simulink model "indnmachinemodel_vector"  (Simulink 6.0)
settings: Solver=ode4  StartTime=0  StopTime=1.2  FixedStep=1e-6  MaxStep=1e-4  RelTol=1e-3  AbsTol=1e-6
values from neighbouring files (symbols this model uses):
  fluxr = 0.2715    [PARAM.M]
  J = 0.0226    [PARAM.M]
  Lm = 4e-3    (= 0.004)    [PARAM.M]
  p = 4    [PARAM.M]
  Rr = .39    (= 0.39)    [PARAM.M]
  Rs = .19    (= 0.19)    [PARAM.M]
  Tr = Lr/Rr    (= 0.0117948717949)    [PARAM.M]
  Vd = 300    [PARAM.M]
  wb = 2*pi*fb    (= 628.318530718)    [PARAM.M]
  Xlr = wb*Llr    (= 0.376991118431)    [PARAM.M]
  Xls = wb*Lls    (= 0.131946891451)    [PARAM.M]
  Xmstar = 1/(1/Xls+1/Xm+1/Xlr)    (= 0.0940797800005)    [PARAM.M]
undefined symbols (not defined in the file or in its folder): magnitude
libraries: simulink x2

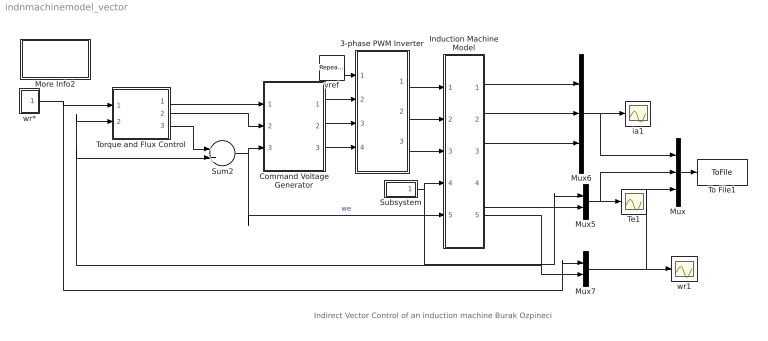
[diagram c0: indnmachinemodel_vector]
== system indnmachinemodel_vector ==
  note: Indirect Vector Control of an induction machine Burak Ozpineci
  3-phase PWM Inverter : Subsystem  PropExecContextAcrossSSBoundary=on
  Command Voltage Generator : Subsystem  PropExecContextAcrossSSBoundary=on
  Induction Machine Model : Subsystem  PropExecContextAcrossSSBoundary=on
  More Info2 : Subsystem  PropExecContextAcrossSSBoundary=on
  Mux : Mux  Inputs=3
  Mux5 : Mux  Inputs=2
  Mux6 : Mux  Inputs=3
  Mux7 : Mux  Inputs=2
  Subsystem : Subsystem  PropExecContextAcrossSSBoundary=on
  Sum2 : Sum
  Te1 : Scope
  To File1 : ToFile  Filename=iemdc2.mat  MatrixName=iemdc
  Torque and Flux Control : Subsystem  PropExecContextAcrossSSBoundary=on
  ia1 : Scope
  vref : simulink/Sources/Repeating Sequence  rep_seq_t=[0 25e-6 50e-6 75e-6 100e-6]  rep_seq_y=[0 1 0 -1 0]
  wr* : Subsystem  PropExecContextAcrossSSBoundary=on
  wr1 : Scope
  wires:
  Induction Machine Model/1(ia) -> Mux6/1
  Induction Machine Model/2(ib) -> Mux6/2
  Induction Machine Model/3(ic) -> Mux6/3
  vref/1 -> 3-phase PWM Inverter/1(vref)
  Torque and Flux Control/3(wsl) -> Sum2/1
  wr*/1(wr*) -> Torque and Flux Control/1(wr*), Mux7/1
  Sum2/1 -> Command Voltage Generator/3(we), Induction Machine Model/5(we)  "we"
  Torque and Flux Control/1(vqs*) -> Command Voltage Generator/1(vqs*)
  Torque and Flux Control/2(vds*) -> Command Voltage Generator/2(vds*)
  Command Voltage Generator/1(vao*) -> 3-phase PWM Inverter/2(vao*)
  Command Voltage Generator/2(vbo*) -> 3-phase PWM Inverter/3(vbo*)
  Command Voltage Generator/3(vco*) -> 3-phase PWM Inverter/4(vco*)
  3-phase PWM Inverter/3(vco) -> Induction Machine Model/3(vco)
  3-phase PWM Inverter/2(vbo) -> Induction Machine Model/2(vbo)
  3-phase PWM Inverter/1(vao) -> Induction Machine Model/1(vao)
  Mux6/1 -> Mux/1, ia1/1
  Induction Machine Model/4(Te) -> Mux5/2
  Mux5/1 -> Mux/2, Te1/1
  Induction Machine Model/5(wr) -> Torque and Flux Control/2(wr), Sum2/2, Mux7/2
  Mux7/1 -> wr1/1, Mux/3
  Subsystem/1(Tl) -> Induction Machine Model/4(Tl), Mux5/1
  Mux/1 -> To File1/1

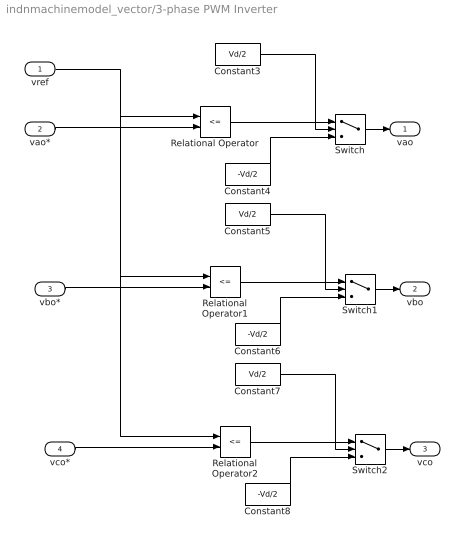
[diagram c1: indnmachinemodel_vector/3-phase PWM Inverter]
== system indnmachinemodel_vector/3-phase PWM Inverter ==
  vref : Inport  LatchInput=off
  vao* : Inport  Port=2  LatchInput=off
  vbo* : Inport  Port=3  LatchInput=off
  vco* : Inport  Port=4  LatchInput=off
  Constant3 : Constant  Value=Vd/2
  Constant4 : Constant  Value=-Vd/2
  Constant5 : Constant  Value=Vd/2
  Constant6 : Constant  Value=-Vd/2
  Constant7 : Constant  Value=Vd/2
  Constant8 : Constant  Value=-Vd/2
  Relational Operator : RelationalOperator  Operator=<=
  Relational Operator1 : RelationalOperator  Operator=<=
  Relational Operator2 : RelationalOperator  Operator=<=
  Switch : Switch  Threshold=0.5
  Switch1 : Switch  Threshold=0.5
  Switch2 : Switch  Threshold=0.5
  vao : Outport
  vbo : Outport  Port=2
  vco : Outport  Port=3
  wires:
  vao*/1 -> Relational Operator/2
  Switch/1 -> vao/1
  Constant4/1 -> Switch/3
  Constant3/1 -> Switch/1
  Relational Operator/1 -> Switch/2
  vbo*/1 -> Relational Operator1/2
  Switch1/1 -> vbo/1
  Constant6/1 -> Switch1/3
  Constant5/1 -> Switch1/1
  vco*/1 -> Relational Operator2/2
  Switch2/1 -> vco/1
  Constant8/1 -> Switch2/3
  Constant7/1 -> Switch2/1
  Relational Operator2/1 -> Switch2/2
  vref/1 -> Relational Operator/1, Relational Operator1/1, Relational Operator2/1
  Relational Operator1/1 -> Switch1/2

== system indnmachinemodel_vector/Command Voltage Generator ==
  vqs* : Inport  LatchInput=off
  vds* : Inport  Port=2  LatchInput=off
  we : Inport  Port=3  LatchInput=off
  Estimator1 : Subsystem  PropExecContextAcrossSSBoundary=on
  Syn-abc3 : Subsystem  PropExecContextAcrossSSBoundary=on
  unit vectors : Subsystem  PropExecContextAcrossSSBoundary=on
  vao* : Outport
  vbo* : Outport  Port=2
  vco* : Outport  Port=3
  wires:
  Syn-abc3/1(vao*) -> vao*/1
  unit vectors/1(cos(theta-e)) -> Syn-abc3/3(cos(theta-e))
  unit vectors/2(sin(theta-e)) -> Syn-abc3/4(sin(theta-e))
  Estimator1/1(theta-e) -> unit vectors/1(theta-e)
  we/1 -> Estimator1/1(we)
  vds*/1 -> Syn-abc3/2(vds)
  vqs*/1 -> Syn-abc3/1(vqs)
  Syn-abc3/2(vbo*) -> vbo*/1
  Syn-abc3/3(vco*) -> vco*/1

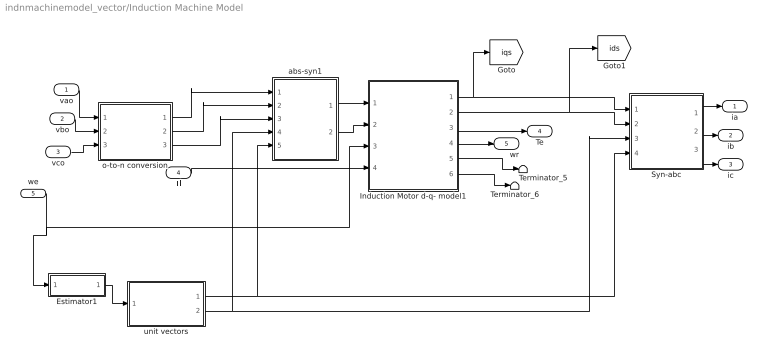
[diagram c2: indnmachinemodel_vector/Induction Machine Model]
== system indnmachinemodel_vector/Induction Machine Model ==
  vao : Inport  LatchInput=off
  vbo : Inport  Port=2  LatchInput=off
  vco : Inport  Port=3  LatchInput=off
  Tl : Inport  Port=4  LatchInput=off
  we : Inport  Port=5  LatchInput=off
  Estimator1 : Subsystem  PropExecContextAcrossSSBoundary=on
  Induction Motor d-q- model1 : Subsystem  PropExecContextAcrossSSBoundary=on
  Syn-abc : Subsystem  PropExecContextAcrossSSBoundary=on
  Terminator_5 : Terminator
  Terminator_6 : Terminator
  abs-syn1 : Subsystem  PropExecContextAcrossSSBoundary=on
  o-to-n conversion : Subsystem  PropExecContextAcrossSSBoundary=on
  unit vectors : Subsystem  PropExecContextAcrossSSBoundary=on
  ia : Outport
  ib : Outport  Port=2
  ic : Outport  Port=3
  Te : Outport  Port=4
  wr : Outport  Port=5
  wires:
  we/1 -> Induction Motor d-q- model1/3(we), Estimator1/1(we)
  Estimator1/1(theta-e) -> unit vectors/1(theta-e)
  Induction Motor d-q- model1/6("iqr ") -> Terminator_6/1
  Tl/1 -> Induction Motor d-q- model1/4(Tl)
  Syn-abc/2(ib) -> ib/1
  Syn-abc/3(ic) -> ic/1
  Induction Motor d-q- model1/5("idr ") -> Terminator_5/1
  Syn-abc/1(ia) -> ia/1
  Induction Motor d-q- model1/3("Te ") -> Te/1
  Induction Motor d-q- model1/4("wr ") -> wr/1
  vao/1 -> o-to-n conversion/1(vao)
  vbo/1 -> o-to-n conversion/2(vbo)
  vco/1 -> o-to-n conversion/3(vco)
  unit vectors/1(sin(theta-e)) -> Syn-abc/4(sin(theta-e)), abs-syn1/5(sin(theta-e))
  unit vectors/2(cos(theta-e)) -> Syn-abc/3(cos(theta-e)), abs-syn1/4(cos(theta-e))
  Induction Motor d-q- model1/2("ids ") -> Syn-abc/2(ids), [ids]
  Induction Motor d-q- model1/1("iqs ") -> [iqs], Syn-abc/1(iqs)
  o-to-n conversion/1(van) -> abs-syn1/1(van)
  o-to-n conversion/2(vbn) -> abs-syn1/2(vbn)
  o-to-n conversion/3(vcn) -> abs-syn1/3(vcn)
  abs-syn1/2(vds) -> Induction Motor d-q- model1/2(vds)
  abs-syn1/1(vqs) -> Induction Motor d-q- model1/1(vqs)

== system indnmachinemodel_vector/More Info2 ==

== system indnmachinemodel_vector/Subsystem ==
  Step2 : Step  Time=.8  After=20  SampleTime=0
  Step3 : Step  After=-10  SampleTime=0
  Step4 : Step  Time=30  After=0  SampleTime=0
  Sum1 : Sum  Inputs=|+++
  Tl : Outport
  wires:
  Step3/1 -> Sum1/2
  Step2/1 -> Sum1/1
  Step4/1 -> Sum1/3
  Sum1/1 -> Tl/1

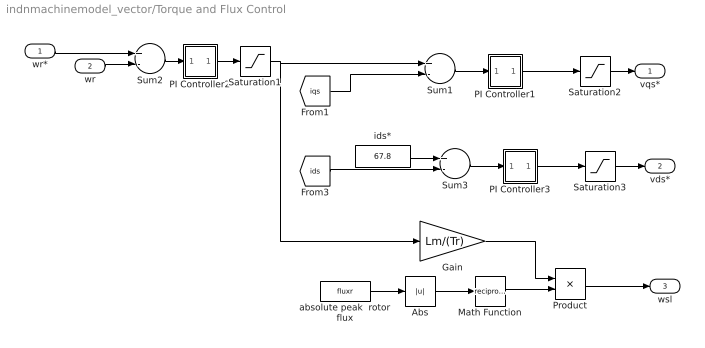
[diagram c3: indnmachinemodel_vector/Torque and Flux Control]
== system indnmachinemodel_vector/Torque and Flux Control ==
  wr* : Inport  LatchInput=off
  wr : Inport  Port=2  LatchInput=off
  Abs : Abs
  Gain : Gain  Gain=Lm/(Tr)
  Math Function : Math  Operator=reciprocal
  PI Controller1 : Subsystem  PropExecContextAcrossSSBoundary=on  mask(PI Controller){P=10000, I=100}
      mask prompts: P "Proportional:"; I "Integral:"
      mask help: Enter expressions for proportional, integral, and derivative terms. P+I/s
  PI Controller2 : Subsystem  PropExecContextAcrossSSBoundary=on  mask(PI Controller){P=500, I=1}
      mask prompts: P "Proportional:"; I "Integral:"
      mask help: Enter expressions for proportional, integral, and derivative terms. P+I/s
  PI Controller3 : Subsystem  PropExecContextAcrossSSBoundary=on  mask(PI Controller){P=1000, I=100}
      mask prompts: P "Proportional:"; I "Integral:"
      mask help: Enter expressions for proportional, integral, and derivative terms. P+I/s
  Product : Product
  Saturation1 : Saturate  UpperLimit=500  LowerLimit=-500
  Saturation2 : Saturate  UpperLimit=1  LowerLimit=-1
  Saturation3 : Saturate  UpperLimit=1  LowerLimit=-1
  Sum1 : Sum  Inputs=+-
  Sum2 : Sum  Inputs=+-
  Sum3 : Sum  Inputs=+-
  absolute peak  rotor flux : Constant  Value=fluxr
  ids* : Constant  Value=67.8
  vqs* : Outport  InitialOutput=0
  vds* : Outport  Port=2  InitialOutput=0
  wsl : Outport  Port=3  InitialOutput=0
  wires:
  absolute peak  rotor flux/1 -> Abs/1
  Gain/1 -> Product/1
  Abs/1 -> Math Function/1
  Math Function/1 -> Product/2
  wr/1 -> Sum2/2
  Sum2/1 -> PI Controller2/1(e)
  wr*/1 -> Sum2/1
  Product/1 -> wsl/1
  Sum1/1 -> PI Controller1/1(e)
  PI Controller2/1(m) -> Saturation1/1
  PI Controller1/1(m) -> Saturation2/1
  Saturation2/1 -> vqs*/1
  Saturation3/1 -> vds*/1
  Sum3/1 -> PI Controller3/1(e)
  PI Controller3/1(m) -> Saturation3/1
  [iqs] -> Sum1/2
  ids*/1 -> Sum3/1
  [ids] -> Sum3/2
  Saturation1/1 -> Gain/1, Sum1/1

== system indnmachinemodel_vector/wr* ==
  Repeating Sequence : simulink/Sources/Repeating Sequence  rep_seq_t=[0 .15 .35 .4 .55 .6 10]  rep_seq_y=[0 .8*wb .8*wb .50*wb .50*wb .65*wb .65*wb]
  wr* : Outport
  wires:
  Repeating Sequence/1 -> wr*/1

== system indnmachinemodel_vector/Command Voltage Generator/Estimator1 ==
  we : Inport  LatchInput=off
  Constant : Constant  Value=2*pi
  Integrator : Integrator  InitialCondition=pi/6
  Math Function3 : Math  Operator=mod
  theta-e : Outport
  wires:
  Math Function3/1 -> theta-e/1
  Integrator/1 -> Math Function3/1
  Constant/1 -> Math Function3/2
  we/1 -> Integrator/1

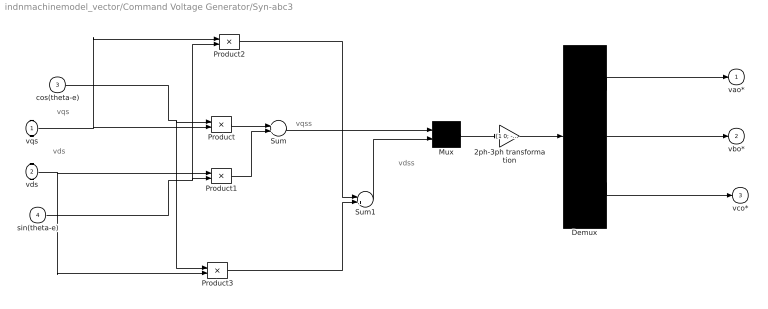
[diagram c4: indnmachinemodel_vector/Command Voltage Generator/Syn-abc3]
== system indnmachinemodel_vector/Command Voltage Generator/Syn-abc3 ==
  note: vqss
  note: vqs
  note: vdss
  note: vds
  vqs : Inport  LatchInput=off
  vds : Inport  Port=2  LatchInput=off
  cos(theta-e) : Inport  Port=3  LatchInput=off
  sin(theta-e) : Inport  Port=4  LatchInput=off
  2ph-3ph transformation : Gain  Gain="[1 0; -1/2 -sqrt(3)/2;  -1/2 sqrt(3)/2]"  Multiplication=Matrix(K*u)
  Demux : Demux  Outputs=3
  Mux : Mux  Inputs=2
  Product{,1..3} (4 alike) : Product
  Sum : Sum
  Sum1 : Sum  Inputs=-+
  vao* : Outport
  vbo* : Outport  Port=2
  vco* : Outport  Port=3
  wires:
  2ph-3ph transformation/1 -> Demux/1
  Sum1/1 -> Mux/2
  Product/1 -> Sum/1
  Product1/1 -> Sum/2
  sin(theta-e)/1 -> Product2/2, Product1/2
  cos(theta-e)/1 -> Product3/1, Product/1
  Product3/1 -> Sum1/2
  Product2/1 -> Sum1/1
  Mux/1 -> 2ph-3ph transformation/1
  vds/1 -> Product3/2, Product1/1
  vqs/1 -> Product2/1, Product/2
  Demux/1 -> vao*/1
  Demux/2 -> vbo*/1
  Demux/3 -> vco*/1
  Sum/1 -> Mux/1

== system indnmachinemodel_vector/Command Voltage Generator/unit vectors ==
  theta-e : Inport  LatchInput=off
  Trigonometric Function : Trigonometry
  Trigonometric Function1 : Trigonometry  Operator=cos
  cos(theta-e) : Outport
  sin(theta-e) : Outport  Port=2
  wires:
  Trigonometric Function/1 -> sin(theta-e)/1
  Trigonometric Function1/1 -> cos(theta-e)/1
  theta-e/1 -> Trigonometric Function1/1, Trigonometric Function/1

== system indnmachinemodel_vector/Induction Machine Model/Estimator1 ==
  we : Inport  LatchInput=off
  Constant : Constant  Value=2*pi
  Integrator : Integrator  InitialCondition=0.01
  Math Function3 : Math  Operator=mod
  theta-e : Outport
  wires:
  we/1 -> Integrator/1
  Constant/1 -> Math Function3/2
  Integrator/1 -> Math Function3/1
  Math Function3/1 -> theta-e/1

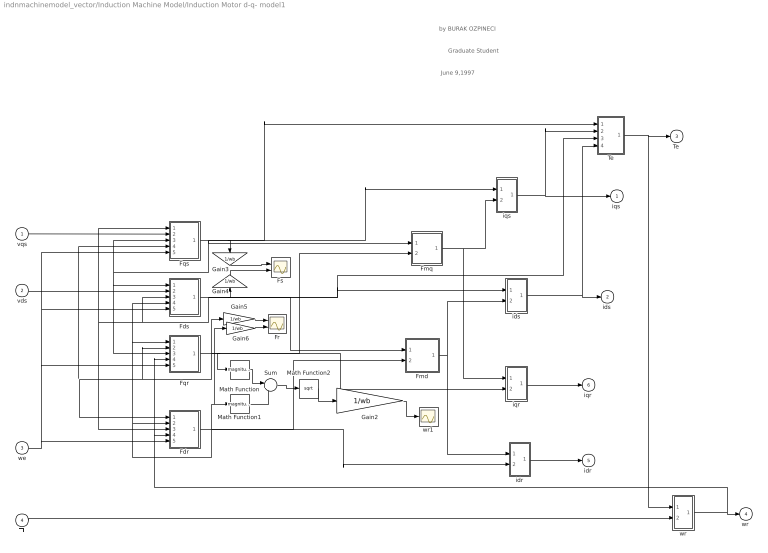
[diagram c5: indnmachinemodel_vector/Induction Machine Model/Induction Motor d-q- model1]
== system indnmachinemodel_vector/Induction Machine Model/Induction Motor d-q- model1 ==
  note: by BURAK OZPINECI
  note: Graduate Student
  note: June 9,1997
  vqs : Inport  LatchInput=off
  vds : Inport  Port=2  LatchInput=off
  we : Inport  Port=3  LatchInput=off
  Tl : Inport  Port=4  LatchInput=off
  Fdr : Subsystem  PropExecContextAcrossSSBoundary=on
  Fds : Subsystem  PropExecContextAcrossSSBoundary=on
  Fmd : Subsystem  PropExecContextAcrossSSBoundary=on
  Fmq : Subsystem  PropExecContextAcrossSSBoundary=on
  Fqr : Subsystem  PropExecContextAcrossSSBoundary=on
  Fqs : Subsystem  PropExecContextAcrossSSBoundary=on
  Fr : Scope  NumInputPorts=2
  Fs : Scope  NumInputPorts=2
  Gain2 : Gain  Gain=1/wb
  Gain3 : Gain  Orientation=down  Gain=1/wb
  Gain4 : Gain  Orientation=up  Gain=1/wb
  Gain5 : Gain  Gain=1/wb
  Gain6 : Gain  Gain=1/wb
  Math Function : Math  Operator=magnitude^2
  Math Function1 : Math  Operator=magnitude^2
  Math Function2 : Math  Operator=sqrt
  Sum : Sum  Inputs=|++
  Te : Subsystem  PropExecContextAcrossSSBoundary=on
  idr : Subsystem  PropExecContextAcrossSSBoundary=on
  ids : Subsystem  PropExecContextAcrossSSBoundary=on
  iqr : Subsystem  PropExecContextAcrossSSBoundary=on
  iqs : Subsystem  PropExecContextAcrossSSBoundary=on
  wr : Subsystem  PropExecContextAcrossSSBoundary=on
  wr1 : Scope
  "iqs " : Outport
  "ids " : Outport  Port=2
  "Te " : Outport  Port=3
  "wr " : Outport  Port=4
  "idr " : Outport  Port=5
  "iqr " : Outport  Port=6
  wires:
  Fdr/1("Fdr ") -> idr/2(Fdr), Fdr/2(Fdr), Fqr/1(Fdr), Fds/4(Fdr), Fmd/2(Fdr), Math Function1/1, Gain6/1
  we/1 -> Fqs/5(we), Fds/5(we), Fqr/5(we), Fdr/5(we)
  wr/1(wr) -> "wr "/1, Fqr/4(wr), Fdr/4(wr)
  vqs/1 -> Fqs/2(Vqs)
  vds/1 -> Fds/2(Vds)
  Tl/1 -> wr/2(Tl)
  Fqs/1("Fqs ") -> Fqs/3(Fqs), Fqr/3(Fqs), Fds/1(Fqs), Fmq/1(Fqs), iqs/1(Fqs), Te/1(Fqs), Gain3/1
  Fqr/1("Fqr ") -> Fqr/2(Fqr), Fqs/4(Fqr), Fdr/1(Fqr), Fmq/2(Fqr), Math Function/1, iqr/2(Fqr), Gain5/1
  Fds/1("Fds ") -> Fds/3(Fds), Fqs/1(Fds), Fdr/3(Fds), Fmd/1(Fds), ids/1(Fds), Te/3(Fds), Gain4/1
  iqr/1(iqr) -> "iqr "/1
  Fmq/1(Fmq) -> iqs/2(Fmq), iqr/1(Fmq)
  idr/1(idr) -> "idr "/1
  Fmd/1(Fmd) -> ids/2(Fmd), idr/1(Fmd)
  Te/1(Te) -> "Te "/1, wr/1(Te)
  ids/1(ids) -> "ids "/1, Te/4(ids)
  iqs/1(iqs) -> "iqs "/1, Te/2(iqs)
  Math Function/1 -> Sum/1
  Math Function1/1 -> Sum/2
  Sum/1 -> Math Function2/1
  Math Function2/1 -> Gain2/1
  Gain2/1 -> wr1/1
  Gain3/1 -> Fs/1
  Gain4/1 -> Fs/2
  Gain5/1 -> Fr/1
  Gain6/1 -> Fr/2

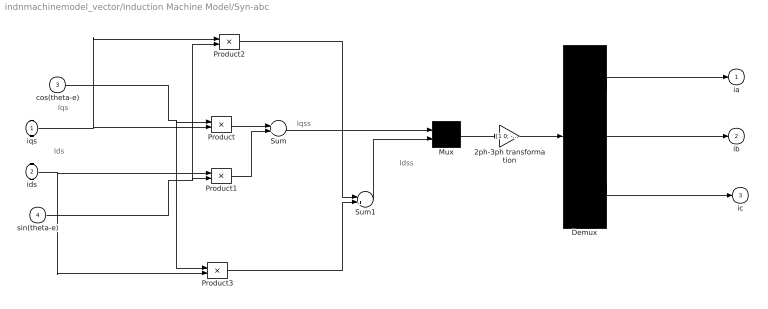
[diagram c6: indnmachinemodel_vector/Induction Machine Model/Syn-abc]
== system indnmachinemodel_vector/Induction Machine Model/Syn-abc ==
  note: Iqss
  note: Iqs
  note: Idss
  note: Ids
  iqs : Inport  LatchInput=off
  ids : Inport  Port=2  LatchInput=off
  cos(theta-e) : Inport  Port=3  LatchInput=off
  sin(theta-e) : Inport  Port=4  LatchInput=off
  2ph-3ph transformation : Gain  Gain="[1 0; -1/2 -sqrt(3)/2;  -1/2 sqrt(3)/2]"  Multiplication=Matrix(K*u)
  Demux : Demux  Outputs=3
  Mux : Mux  Inputs=2
  Product{,1..3} (4 alike) : Product
  Sum : Sum
  Sum1 : Sum  Inputs=-+
  ia : Outport
  ib : Outport  Port=2
  ic : Outport  Port=3
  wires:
  2ph-3ph transformation/1 -> Demux/1
  Sum1/1 -> Mux/2
  Sum/1 -> Mux/1
  Product/1 -> Sum/1
  Product1/1 -> Sum/2
  sin(theta-e)/1 -> Product2/2, Product1/2
  cos(theta-e)/1 -> Product3/1, Product/1
  Product3/1 -> Sum1/2
  Product2/1 -> Sum1/1
  Mux/1 -> 2ph-3ph transformation/1
  ids/1 -> Product3/2, Product1/1
  iqs/1 -> Product2/1, Product/2
  Demux/1 -> ia/1
  Demux/2 -> ib/1
  Demux/3 -> ic/1

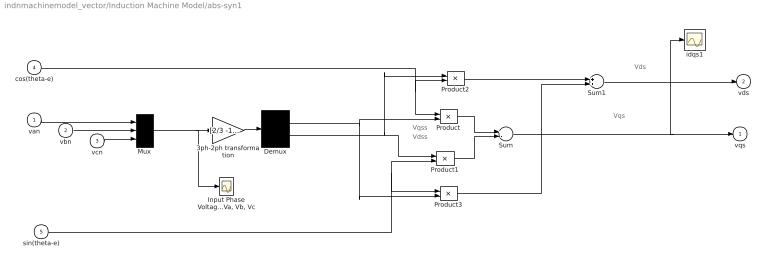
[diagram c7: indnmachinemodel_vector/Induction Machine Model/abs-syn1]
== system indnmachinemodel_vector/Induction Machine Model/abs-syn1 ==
  note: Vqs
  note: Vds
  note: Vqss
  note: Vdss
  van : Inport  LatchInput=off
  vbn : Inport  Port=2  LatchInput=off
  vcn : Inport  Port=3  LatchInput=off
  cos(theta-e) : Inport  Port=4  LatchInput=off
  sin(theta-e) : Inport  Port=5  LatchInput=off
  3ph-2ph transformation : Gain  Gain=[2/3 -1/3 -1/3;0 -1/sqrt(3) 1/sqrt(3)]  Multiplication=Matrix(K*u)
  Demux : Demux  Outputs=2
  "Input Phase Voltages Va, Vb, Vc" : Scope
  Mux : Mux  Inputs=3
  Product{,1..3} (4 alike) : Product
  Sum : Sum  Inputs=+-
  Sum1 : Sum
  idqs1 : Scope
  vqs : Outport
  vds : Outport  Port=2
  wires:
  cos(theta-e)/1 -> Product2/2, Product/1
  sin(theta-e)/1 -> Product3/1, Product1/2
  Demux/1 -> Product3/2, Product/2
  van/1 -> Mux/1
  Demux/2 -> Product1/1, Product2/1
  vbn/1 -> Mux/2
  Product3/1 -> Sum1/2
  Product2/1 -> Sum1/1
  Sum/1 -> idqs1/1, vqs/1
  Sum1/1 -> vds/1
  Product1/1 -> Sum/2
  Mux/1 -> 3ph-2ph transformation/1, "Input Phase Voltages Va, Vb, Vc"/1
  vcn/1 -> Mux/3
  Product/1 -> Sum/1
  3ph-2ph transformation/1 -> Demux/1

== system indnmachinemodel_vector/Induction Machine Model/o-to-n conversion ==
  vao : Inport  LatchInput=off
  vbo : Inport  Port=2  LatchInput=off
  vco : Inport  Port=3  LatchInput=off
  Demux : Demux  Outputs=3
  Matrix Gain : Gain  Gain=[2/3 -1/3 -1/3; -1/3 2/3 -1/3; -1/3 -1/3 2/3]  Multiplication=Matrix(K*u)
  Mux : Mux  Inputs=3
  van : Outport
  vbn : Outport  Port=2
  vcn : Outport  Port=3
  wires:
  Demux/3 -> vcn/1
  Demux/2 -> vbn/1
  Demux/1 -> van/1
  vco/1 -> Mux/3
  vbo/1 -> Mux/2
  vao/1 -> Mux/1
  Matrix Gain/1 -> Demux/1
  Mux/1 -> Matrix Gain/1

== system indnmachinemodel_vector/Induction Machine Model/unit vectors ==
  theta-e : Inport  LatchInput=off
  Trigonometric Function : Trigonometry
  Trigonometric Function1 : Trigonometry  Operator=cos
  sin(theta-e) : Outport
  cos(theta-e) : Outport  Port=2
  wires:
  theta-e/1 -> Trigonometric Function/1, Trigonometric Function1/1
  Trigonometric Function1/1 -> cos(theta-e)/1
  Trigonometric Function/1 -> sin(theta-e)/1

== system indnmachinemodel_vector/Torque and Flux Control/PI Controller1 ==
  e : Inport  LatchInput=off
  Integral : TransferFcn  Numerator=[I]  Denominator=[1 0]
  Proportional : Gain  Gain=P
  Sum : Sum
  m : Outport  InitialOutput=0
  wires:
  e/1 -> Proportional/1, Integral/1
  Sum/1 -> m/1
  Integral/1 -> Sum/2
  Proportional/1 -> Sum/1

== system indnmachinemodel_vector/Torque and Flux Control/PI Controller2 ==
  e : Inport  LatchInput=off
  Integral : TransferFcn  Numerator=[I]  Denominator=[1 0]
  Proportional : Gain  Gain=P
  Sum : Sum
  m : Outport  InitialOutput=0
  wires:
  e/1 -> Proportional/1, Integral/1
  Sum/1 -> m/1
  Integral/1 -> Sum/2
  Proportional/1 -> Sum/1

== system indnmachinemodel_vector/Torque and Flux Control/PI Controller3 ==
  e : Inport  LatchInput=off
  Integral : TransferFcn  Numerator=[I]  Denominator=[1 0]
  Proportional : Gain  Gain=P
  Sum : Sum
  m : Outport  InitialOutput=0
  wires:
  Proportional/1 -> Sum/1
  Integral/1 -> Sum/2
  Sum/1 -> m/1
  e/1 -> Integral/1, Proportional/1

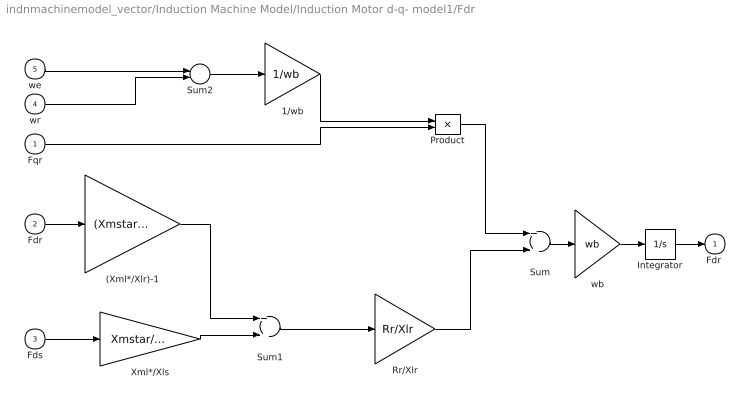
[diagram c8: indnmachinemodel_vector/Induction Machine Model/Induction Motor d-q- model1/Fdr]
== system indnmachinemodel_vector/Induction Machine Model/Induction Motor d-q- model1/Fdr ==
  Fqr : Inport  LatchInput=off
  Fdr : Inport  Port=2  LatchInput=off
  Fds : Inport  Port=3  LatchInput=off
  wr : Inport  Port=4  LatchInput=off
  we : Inport  Port=5  LatchInput=off
  (Xml*/Xlr)-1 : Gain  Gain=(Xmstar/Xlr)-1
  1/wb : Gain  Gain=1/wb
  Integrator : Integrator
  Product : Product
  Rr/Xlr : Gain  Gain=Rr/Xlr
  Sum : Sum
  Sum1 : Sum
  Sum2 : Sum  Inputs=+-
  Xml*/Xls : Gain  Gain=Xmstar/Xls
  wb : Gain  Gain=wb
  "Fdr " : Outport
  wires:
  Rr/Xlr/1 -> Sum/2
  Xml*/Xls/1 -> Sum1/2
  (Xml*/Xlr)-1/1 -> Sum1/1
  Product/1 -> Sum/1
  1/wb/1 -> Product/1
  wr/1 -> Sum2/2
  Fqr/1 -> Product/2
  we/1 -> Sum2/1
  Sum2/1 -> 1/wb/1
  Fds/1 -> Xml*/Xls/1
  Integrator/1 -> "Fdr "/1
  Fdr/1 -> (Xml*/Xlr)-1/1
  Sum1/1 -> Rr/Xlr/1
  Sum/1 -> wb/1
  wb/1 -> Integrator/1

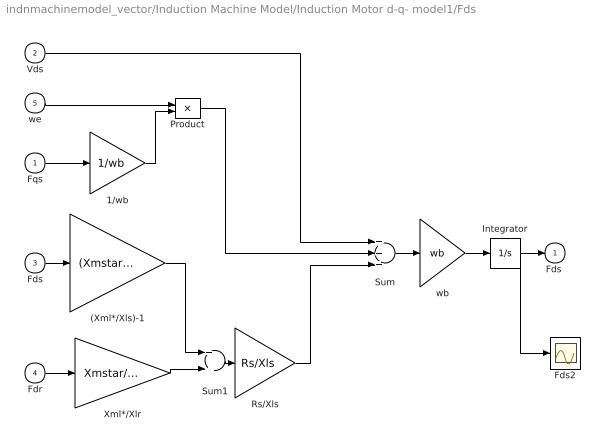
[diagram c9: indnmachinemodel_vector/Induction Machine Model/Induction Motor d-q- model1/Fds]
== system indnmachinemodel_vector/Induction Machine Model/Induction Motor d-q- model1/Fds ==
  Fqs : Inport  LatchInput=off
  Vds : Inport  Port=2  LatchInput=off
  Fds : Inport  Port=3  LatchInput=off
  Fdr : Inport  Port=4  LatchInput=off
  we : Inport  Port=5  LatchInput=off
  (Xml*/Xls)-1 : Gain  Gain=(Xmstar/Xls)-1
  1/wb : Gain  Gain=1/wb
  Fds2 : Scope
  Integrator : Integrator
  Product : Product
  Rs/Xls : Gain  Gain=Rs/Xls
  Sum : Sum  Inputs=+++
  Sum1 : Sum
  Xml*/Xlr : Gain  Gain=Xmstar/Xlr
  wb : Gain  Gain=wb
  "Fds " : Outport
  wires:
  1/wb/1 -> Product/2
  Product/1 -> Sum/2
  we/1 -> Product/1
  wb/1 -> Integrator/1
  Fdr/1 -> Xml*/Xlr/1
  Fds/1 -> (Xml*/Xls)-1/1
  Vds/1 -> Sum/1
  Fqs/1 -> 1/wb/1
  Rs/Xls/1 -> Sum/3
  (Xml*/Xls)-1/1 -> Sum1/1
  Xml*/Xlr/1 -> Sum1/2
  Sum1/1 -> Rs/Xls/1
  Sum/1 -> wb/1
  Integrator/1 -> "Fds "/1, Fds2/1

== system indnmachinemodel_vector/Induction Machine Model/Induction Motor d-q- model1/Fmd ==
  Fds : Inport  LatchInput=off
  Fdr : Inport  Port=2  LatchInput=off
  Sum8 : Sum
  Xmstar/Xlr : Gain  Gain=Xmstar/Xlr
  Xmstar/Xls : Gain  Gain=Xmstar/Xls
  Fmd : Outport
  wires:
  Fdr/1 -> Xmstar/Xlr/1
  Sum8/1 -> Fmd/1
  Fds/1 -> Xmstar/Xls/1
  Xmstar/Xls/1 -> Sum8/1
  Xmstar/Xlr/1 -> Sum8/2

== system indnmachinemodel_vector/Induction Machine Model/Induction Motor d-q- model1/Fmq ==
  Fqs : Inport  LatchInput=off
  Fqr : Inport  Port=2  LatchInput=off
  Sum8 : Sum
  Xmstar/Xlr : Gain  Gain=Xmstar/Xlr
  Xmstar/Xls : Gain  Gain=Xmstar/Xls
  Fmq : Outport
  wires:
  Fqr/1 -> Xmstar/Xlr/1
  Sum8/1 -> Fmq/1
  Fqs/1 -> Xmstar/Xls/1
  Xmstar/Xls/1 -> Sum8/1
  Xmstar/Xlr/1 -> Sum8/2

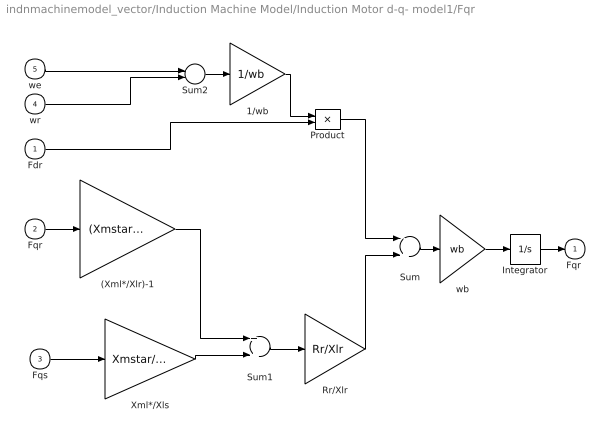
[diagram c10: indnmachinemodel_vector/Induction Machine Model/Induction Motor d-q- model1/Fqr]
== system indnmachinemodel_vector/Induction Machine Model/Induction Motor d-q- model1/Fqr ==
  Fdr : Inport  LatchInput=off
  Fqr : Inport  Port=2  LatchInput=off
  Fqs : Inport  Port=3  LatchInput=off
  wr : Inport  Port=4  LatchInput=off
  we : Inport  Port=5  LatchInput=off
  (Xml*/Xlr)-1 : Gain  Gain=(Xmstar/Xlr)-1
  1/wb : Gain  Gain=1/wb
  Integrator : Integrator
  Product : Product
  Rr/Xlr : Gain  Gain=Rr/Xlr
  Sum : Sum  Inputs=-+
  Sum1 : Sum
  Sum2 : Sum  Inputs=+-
  Xml*/Xls : Gain  Gain=Xmstar/Xls
  wb : Gain  Gain=wb
  "Fqr " : Outport
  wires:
  (Xml*/Xlr)-1/1 -> Sum1/1
  Rr/Xlr/1 -> Sum/2
  Product/1 -> Sum/1
  Fdr/1 -> Product/2
  1/wb/1 -> Product/1
  Sum2/1 -> 1/wb/1
  wr/1 -> Sum2/2
  we/1 -> Sum2/1
  Fqs/1 -> Xml*/Xls/1
  Integrator/1 -> "Fqr "/1
  Fqr/1 -> (Xml*/Xlr)-1/1
  Xml*/Xls/1 -> Sum1/2
  Sum1/1 -> Rr/Xlr/1
  Sum/1 -> wb/1
  wb/1 -> Integrator/1

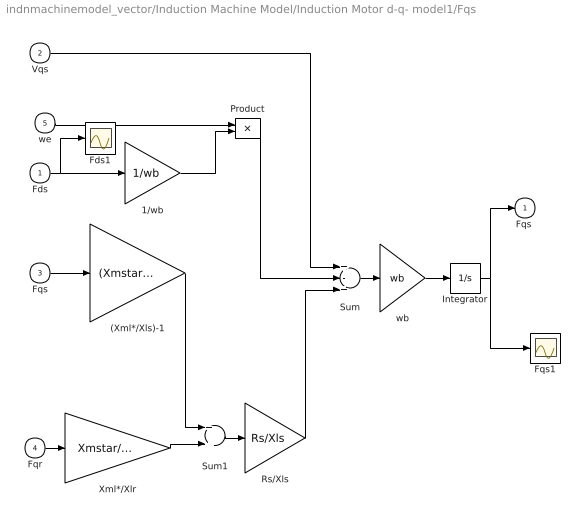
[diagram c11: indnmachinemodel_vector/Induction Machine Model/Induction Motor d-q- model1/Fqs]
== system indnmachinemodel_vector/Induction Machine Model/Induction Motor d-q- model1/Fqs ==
  Fds : Inport  LatchInput=off
  Vqs : Inport  Port=2  LatchInput=off
  Fqs : Inport  Port=3  LatchInput=off
  Fqr : Inport  Port=4  LatchInput=off
  we : Inport  Port=5  LatchInput=off
  (Xml*/Xls)-1 : Gain  Gain=(Xmstar/Xls)-1
  1/wb : Gain  Gain=1/wb
  Fds1 : Scope
  Fqs1 : Scope
  Integrator : Integrator
  Product : Product
  Rs/Xls : Gain  Gain=Rs/Xls
  Sum : Sum  Inputs=+-+
  Sum1 : Sum
  Xml*/Xlr : Gain  Gain=Xmstar/Xlr
  wb : Gain  Gain=wb
  "Fqs " : Outport
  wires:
  1/wb/1 -> Product/2
  Product/1 -> Sum/2
  we/1 -> Product/1
  Xml*/Xlr/1 -> Sum1/2
  (Xml*/Xls)-1/1 -> Sum1/1
  wb/1 -> Integrator/1
  Fqr/1 -> Xml*/Xlr/1
  Fqs/1 -> (Xml*/Xls)-1/1
  Vqs/1 -> Sum/1
  Rs/Xls/1 -> Sum/3
  Sum1/1 -> Rs/Xls/1
  Sum/1 -> wb/1
  Integrator/1 -> "Fqs "/1, Fqs1/1
  Fds/1 -> 1/wb/1, Fds1/1

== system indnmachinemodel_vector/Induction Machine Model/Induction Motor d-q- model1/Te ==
  Fqs : Inport  LatchInput=off
  iqs : Inport  Port=2  LatchInput=off
  Fds : Inport  Port=3  LatchInput=off
  ids : Inport  Port=4  LatchInput=off
  3*p/(4*wb) : Gain  Gain=3*p/(4*wb)
  Product : Product
  Product1 : Product
  Sum7 : Sum  Inputs=+-
  Te : Outport
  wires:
  ids/1 -> Product/2
  Fqs/1 -> Product/1
  iqs/1 -> Product1/2
  Fds/1 -> Product1/1
  3*p/(4*wb)/1 -> Te/1
  Sum7/1 -> 3*p/(4*wb)/1
  Product1/1 -> Sum7/1
  Product/1 -> Sum7/2

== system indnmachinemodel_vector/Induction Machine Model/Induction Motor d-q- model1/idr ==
  Fmd : Inport  LatchInput=off
  Fdr : Inport  Port=2  LatchInput=off
  1/Xlr : Gain  Gain=1/Xlr
  Sum8 : Sum  Inputs=+-
  idr : Outport
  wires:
  Fmd/1 -> Sum8/2
  1/Xlr/1 -> idr/1
  Fdr/1 -> Sum8/1
  Sum8/1 -> 1/Xlr/1

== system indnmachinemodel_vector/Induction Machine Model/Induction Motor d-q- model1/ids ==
  Fds : Inport  LatchInput=off
  Fmd : Inport  Port=2  LatchInput=off
  1/Xls : Gain  Gain=1/Xls
  Sum8 : Sum  Inputs=+-
  ids : Outport
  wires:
  Fmd/1 -> Sum8/2
  1/Xls/1 -> ids/1
  Fds/1 -> Sum8/1
  Sum8/1 -> 1/Xls/1

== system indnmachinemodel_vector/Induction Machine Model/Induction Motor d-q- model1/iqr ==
  Fmq : Inport  LatchInput=off
  Fqr : Inport  Port=2  LatchInput=off
  1/Xlr : Gain  Gain=1/Xlr
  Sum8 : Sum  Inputs=+-
  iqr : Outport
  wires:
  Fmq/1 -> Sum8/2
  1/Xlr/1 -> iqr/1
  Fqr/1 -> Sum8/1
  Sum8/1 -> 1/Xlr/1

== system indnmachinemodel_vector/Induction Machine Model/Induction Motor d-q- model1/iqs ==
  Fqs : Inport  LatchInput=off
  Fmq : Inport  Port=2  LatchInput=off
  1/Xls : Gain  Gain=1/Xls
  Sum8 : Sum  Inputs=+-
  iqs : Outport
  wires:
  Fmq/1 -> Sum8/2
  1/Xls/1 -> iqs/1
  Fqs/1 -> Sum8/1
  Sum8/1 -> 1/Xls/1

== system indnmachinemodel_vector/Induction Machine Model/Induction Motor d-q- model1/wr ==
  Te : Inport  LatchInput=off
  Tl : Inport  Port=2  LatchInput=off
  Integrator : Integrator
  Sum7 : Sum  Inputs=+-
  p/(2*J) : Gain  Gain=p/(2*J)
  wr : Outport
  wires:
  Te/1 -> Sum7/1
  Tl/1 -> Sum7/2
  Integrator/1 -> wr/1
  p/(2*J)/1 -> Integrator/1
  Sum7/1 -> p/(2*J)/1
